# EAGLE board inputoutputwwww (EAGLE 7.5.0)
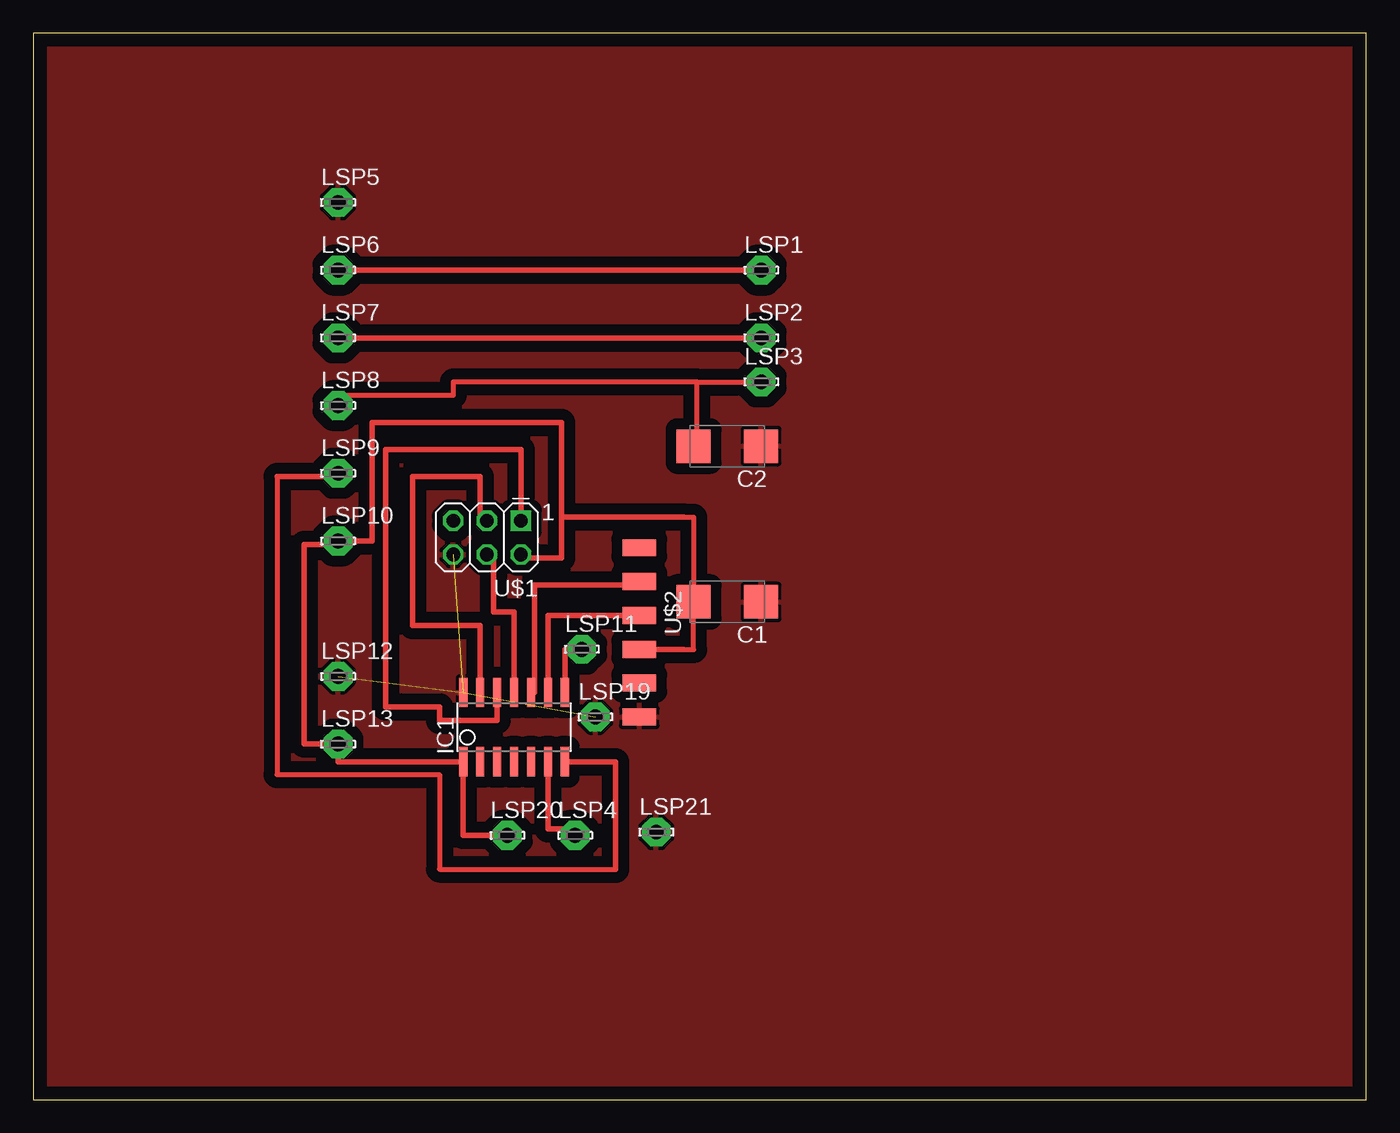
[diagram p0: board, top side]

Size 100 x 80 mm. Coordinates in mm from the lower left corner, seen from the top.
Outline: 0,0 100,0 100,80 0,80 0,0
Copper layers (1*16): Top 0.035mm / dielectric 1.5mm / Bottom 0.035mm
Design rules "default *": minimum track width 10mil, minimum drill 24mil, track to track 16mil, track to pad 16mil, pad to pad 16mil, via to via 16mil, smd to smd 16mil, copper to edge 40mil, drill to drill 8mil, minimum pad ring 10mil, minimum via ring 8mil, stop-mask expansion 4mil, vias tented up to drill 0mil, thermal gap 10mil

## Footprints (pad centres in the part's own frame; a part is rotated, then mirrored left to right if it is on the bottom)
C/6032-28R = smd 2.55 x 2.5: + 2.525,0; - -2.525,0
SOIC14 = smd 0.61 x 2.21: 1 -3.81,-2.603; 2 -2.54,-2.603; 3 -1.27,-2.603; 4 0,-2.603; 5 1.27,-2.603; 6 2.54,-2.603; 7 3.81,-2.603; 8 3.81,2.603; 9 2.54,2.603; 10 1.27,2.603; 11 0,2.603; 12 -1.27,2.603; 13 -2.54,2.603; 14 -3.81,2.603
LSP11 = drill 1.118 pad 2.159 octagon: MP 0,0
2X03 = drill 1.016 square: 1 -2.54,-1.27 | drill 1.016 octagon: 2 -2.54,1.27; 3 0,-1.27; 4 0,1.27; 5 2.54,-1.27; 6 2.54,1.27
1X06SMD = smd 2.54 x 1.27: 1 0,6.35; 2 0,3.81; 3 0,1.27; 4 0,-1.27; 5 0,-3.81; 6 0,-6.35

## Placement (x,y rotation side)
C1  2.2u  [C/6032-28R]  52.07,37.34 180 top
C2  2.2u  [C/6032-28R]  52.07,49.02 180 top
IC1  ATTINY44-SSU  [SOIC14]  36.07,27.94 0 top
LSP1  LSP11  [LSP11]  54.61,62.23 0 top
LSP2  LSP11  [LSP11]  54.61,57.15 0 top
LSP3  LSP11  [LSP11]  54.61,53.85 0 top
LSP4  LSP11  [LSP11]  40.64,19.81 0 top
LSP5  LSP11  [LSP11]  22.86,67.31 0 top
LSP6  LSP11  [LSP11]  22.86,62.23 0 top
LSP7  LSP11  [LSP11]  22.86,57.15 0 top
LSP8  LSP11  [LSP11]  22.86,52.07 0 top
LSP9  LSP11  [LSP11]  22.86,46.99 0 top
LSP10  LSP11  [LSP11]  22.86,41.91 0 top
LSP11  LSP11  [LSP11]  41.15,33.78 0 top
LSP12  LSP11  [LSP11]  22.86,31.75 0 top
LSP13  LSP11  [LSP11]  22.86,26.67 0 top
LSP19  LSP11  [LSP11]  42.16,28.7 0 top
LSP20  LSP11  [LSP11]  35.56,19.81 0 top
LSP21  LSP11  [LSP11]  46.74,20.07 0 top
U$1  AVRISP  [2X03]  34.04,42.16 180 top
U$2  FTDI-SMD-HEADER  [1X06SMD]  45.47,35.05 180 top

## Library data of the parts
C1 C2 = rcl
IC1 U$1 U$2 = fab
LSP1-LSP13 LSP19-LSP21 = solpad

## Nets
+5V: C1.+ IC1.1 LSP10.MP LSP13.MP LSP20.MP U$1.2 U$2.3
GND: C1.- C2.- IC1.14 LSP5.MP LSP12.MP LSP19.MP LSP21.MP U$1.6 U$2.1
IN2: IC1.8 LSP11.MP
N$1: IC1.7 LSP9.MP
N$2: C2.+ LSP3.MP LSP8.MP
N$3: IC1.6 LSP4.MP
N$4: U$1.5
N$5: IC1.13 U$1.3
N$6: IC1.12 U$1.1
N$7: IC1.11 U$1.4
N$8: IC1.9 U$2.4
N$9: IC1.10 U$2.5
OUT1: LSP1.MP LSP6.MP
OUT2: LSP2.MP LSP7.MP

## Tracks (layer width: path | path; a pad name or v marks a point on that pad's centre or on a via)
+5V
  Top 0.37: 48.77,33.77 49.55,33.77 C1.+ 49.55,43.69 48.77,43.69
  Top 0.406: 39.62,43.69 39.62,50.8 25.4,50.8 25.4,41.91 LSP10.MP 22.86,41.66 20.32,41.66 20.32,26.67 LSP13.MP 22.86,25.34 IC1.1 32.26,19.81 LSP20.MP | 39.62,43.69 39.62,40.64 36.58,40.64 U$1.2 | 48.77,43.69 39.62,43.69 | 48.77,33.77 45.47,33.77 U$2.3
_OUTLINES_
  pour Top (isolate 0.825, rank 6): 0,0 100,0 100,80 0,80
GND  (3 unrouted)
  pour Top (isolate 0.825, rank 6): 20.32,70.1 57.91,70.1 57.91,31.5 50.8,31.5 50.8,14.22 28.45,14.22 28.45,22.35 15.24,22.35 15.24,64.01 20.32,64.01
IN2
  Top 0.406: LSP11.MP 39.88,33.78 IC1.8
N$1
  Top 0.37: 18.29,46.74 18.29,24.38 30.48,24.38 30.48,17.27 43.69,17.27
  Top 0.406: IC1.7 43.69,25.34 43.69,17.27 | 18.29,46.74 22.86,46.74 LSP9.MP
N$2
  Top 0.37: 49.78,53.85 LSP3.MP | C2.+ 49.78,49.02 49.78,53.85 | 49.78,53.85 31.5,53.85 31.5,52.83 22.86,52.83 LSP8.MP
N$3
  Top 0.406: IC1.6 38.61,20.32 40.64,20.32 LSP4.MP
N$5
  Top 0.406: U$1.3 33.53,43.43 33.53,46.74 28.45,46.74 28.45,35.56 33.53,35.56 IC1.13
N$6
  Top 0.406: U$1.1 36.58,48.77 26.42,48.77 26.42,29.46 30.48,29.46 30.48,28.45 34.8,28.45 IC1.12
N$7
  Top 0.406: U$1.4 34.54,40.89 34.54,36.58 36.07,36.58 IC1.11
N$8
  Top 0.406: U$2.4 38.61,36.32 IC1.9
N$9
  Top 0.406: IC1.10 37.59,30.54 37.59,38.61 44.45,38.61 U$2.5
OUT1
  Top 0.406: LSP6.MP LSP1.MP
OUT2
  Top 0.406: LSP2.MP LSP7.MP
